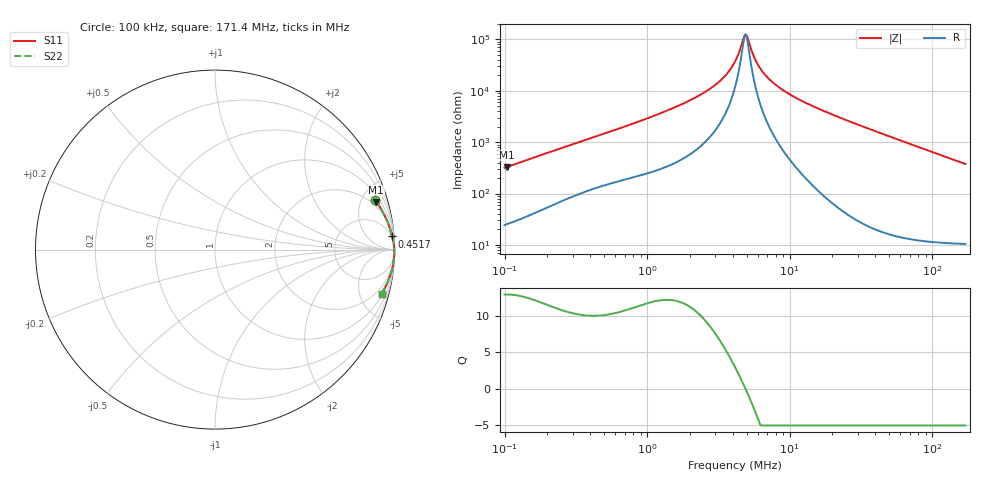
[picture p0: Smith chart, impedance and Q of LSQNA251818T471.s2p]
! LSQNA251818T471  S-PARAMETER MODEL  ( General Type )
! Model Generated by TAIYO YUDEN Corporation (http://www.ty-top.com)
! Version 2.0
! TAIYO YUDEN Control No. 100810NF25SB-FKC
! Copyright(c) 2007 TAIYO YUDEN CO.,LTD. All Rights Reserved.
! Product Description (link to TY-COMPAS)
! https://ds.yuden.co.jp/TYCOMPAS/or/detail?pn=LSQNA251818T471K&u=M
! Products Name : Inductors
! Characteristics :
!  Inductance : 470 uH , SRF(min) : 3.5 MHz , DC Resistance(max) : 13 Ohm
!  Rated Current : Saturation :35 mA , Temp Rise : 120 mA (40 degC)
!  Case Size : 2.5 x 1.8 / 0.098 x 0.071 [mm/inch] , Thickness : 1.8 / 0.071 [mm/inch]
!  (Conditions: Temperature = 25 degC , DC Bias Current/Voltage = 0A / 0V)
! External Node Assignments :
!  1  o---GGG---o  2
! GND o---------o GND
! Frequency Range : 0.1MHz  -  171.398534MHz  [ 402 STEP ]
# MHz S RI R 50
! Freq[MHz].  S11 Real  S11 Imag  S21 Real  S21 Imag  S12 Real  S12 Imag  S22 Real  S22 Imag
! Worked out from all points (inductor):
!   401 points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, 100 kHz to 171.4 MHz, reference 50 ohm
!   read as one part in series: L = 500 uH near 103.8 kHz
!   highest Q = 12.9 at 103.8 kHz (marker M1), where L = 503 uH
!   self-resonance near 4.895 MHz
!   S11 on the Smith chart (normalised r, x): 100 kHz: 1.49, +6.33; 451.7 kHz: 4, +27; 171.4 MHz: 1.21, -7.53
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0.1  0.8924 0.2736  0.1076 -0.2736  0.1076 -0.2736  0.8924 0.2736
0.103793  0.8985 0.2659  0.1015 -0.2659  0.1015 -0.2659  0.8985 0.2659
0.348094  0.982 0.0926  0.018 -0.0926  0.018 -0.0926  0.982 0.0926
0.451738  0.9872 0.0731  0.0128 -0.0731  0.0128 -0.0731  0.9872 0.0731
1.211692  0.9969 0.0278  0.00308 -0.0278  0.00308 -0.0278  0.9969 0.0278
1.966087  0.9984 0.0155  0.00161 -0.0155  0.00161 -0.0155  0.9984 0.0155
2.748737  0.9989 0.00913  0.00114 -0.00913  0.00114 -0.00913  0.9989 0.00913
3.501373  0.9991 0.00514  0.000947 -0.00514  0.000947 -0.00514  0.9991 0.00514
3.842939  0.9991 0.0037  0.000894 -0.0037  0.000894 -0.0037  0.9991 0.0037
4.140031  0.9991 0.00256  0.000859 -0.00256  0.000859 -0.00256  0.9991 0.00256
4.377827  0.9992 0.00172  0.000836 -0.00172  0.000836 -0.00172  0.9992 0.00172
4.804893  0.9992 0.000327  0.000803 -0.000327  0.000803 -0.000327  0.9992 0.000327
4.987165  0.9992 -0.00023  0.000792 0.00023  0.000792 0.00023  0.9992 -0.00023
5.176352  0.9992 -0.000787  0.000782 0.000787  0.000782 0.000787  0.9992 -0.000787
5.576527  0.9992 -0.00191  0.000764 0.00191  0.000764 0.00191  0.9992 -0.00191
5.896834  0.9992 -0.00275  0.000754 0.00275  0.000754 0.00275  0.9992 -0.00275
6.352709  0.9993 -0.0039  0.000743 0.0039  0.000743 0.0039  0.9993 -0.0039
6.972428  0.9993 -0.00536  0.000734 0.00536  0.000734 0.00536  0.9993 -0.00536
9.391703  0.9993 -0.0104  0.000749 0.0104  0.000749 0.0104  0.9993 -0.0104
14.41119  0.9991 -0.0196  0.000947 0.0196  0.000947 0.0196  0.9991 -0.0196
50.16444  0.9932 -0.0764  0.00683 0.0764  0.00683 0.0764  0.9932 -0.0764
171.3985  0.9282 -0.2447  0.0718 0.2447  0.0718 0.2447  0.9282 -0.2447
